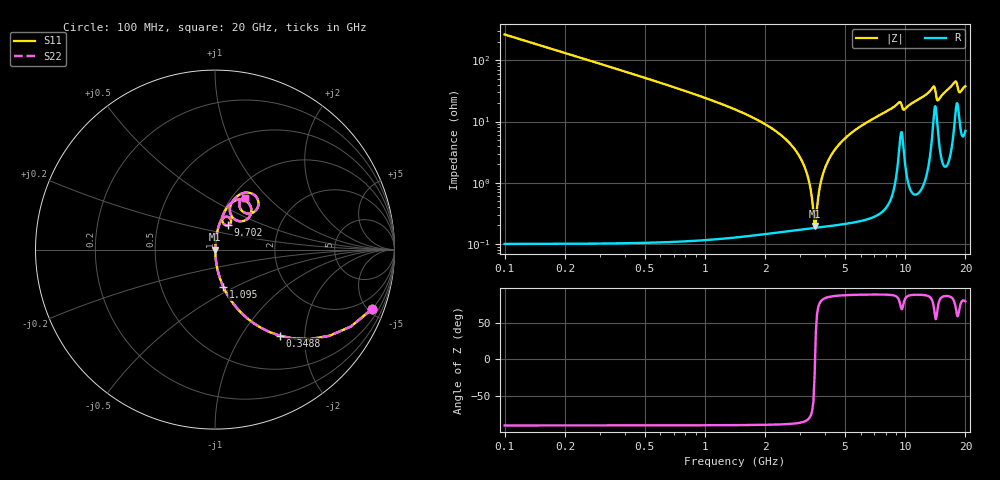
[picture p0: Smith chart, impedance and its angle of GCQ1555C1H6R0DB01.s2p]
!Murata Part Number: GCQ1555C1H6R0DB01
!These Parameters are Measured in Series Mode Connection
!Data Generated on Jan 08, 2026
!  o--ll--o
!Port1  Port2
!  o------o
!Operation Temp=25[degC], DC Bias Voltage=0[V]
!Freq. Start=100[MHz] Stop=20[GHz] 401[Steps]
# Hz S RI R 50
!Freq.(Hz) S11(Real) S11(Imag) S21(Real) S21(Imag) S12(Real) S12(Imag) S22(Real) S22(Imag)
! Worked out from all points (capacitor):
!   401 points, 100 MHz to 20 GHz, reference 50 ohm
!   read as one part in series: C = 6 pF near 199.5 MHz
!   lowest |Z| = 196 mohm at 3.533 GHz (marker M1)
!   series resonance near 3.55 GHz, so ESL is about 340 pH
!   S11 on the Smith chart (normalised r, x): 100 MHz: 1.00, -5.30; 348.8 MHz: 1.00, -1.51; 1.095 GHz: 1.00, -0.44; 9.702 GHz: 1.11, +0.31; 20 GHz: 1.14, +0.74
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1e8  0.8753 -0.3302  0.1247 0.3302  0.1247 0.3302  0.8753 -0.3302
3.4875e8  0.3621 -0.4799  0.6379 0.4799  0.6379 0.4799  0.3621 -0.4799
6.4725e8  0.1363 -0.3418  0.8637 0.3418  0.8637 0.3418  0.1363 -0.3418
1.095e9  0.0468 -0.2086  0.9532 0.2086  0.9532 0.2086  0.0468 -0.2086
2.83625e9  0.0028 -0.0337  0.9972 0.0337  0.9972 0.0337  0.0028 -0.0337
3.23425e9  0.00195 -0.0139  0.9981 0.0139  0.9981 0.0139  0.00195 -0.0139
3.43325e9  0.00182 -0.00498  0.9982 0.00498  0.9982 0.00498  0.00182 -0.00498
3.53275e9  0.00182 -0.000717  0.9982 0.000717  0.9982 0.000717  0.00182 -0.000717
3.63225e9  0.00185 0.00343  0.9982 -0.00343  0.9982 -0.00343  0.00185 0.00343
3.93075e9  0.00213 0.0153  0.9979 -0.0153  0.9979 -0.0153  0.00213 0.0153
4.3785e9  0.00299 0.0316  0.997 -0.0316  0.997 -0.0316  0.00299 0.0316
6.7665e9  0.0137 0.1047  0.9863 -0.1047  0.9863 -0.1047  0.0137 0.1047
9.30375e9  0.065 0.1831  0.935 -0.1831  0.935 -0.1831  0.065 0.1831
9.70175e9  0.073 0.1364  0.927 -0.1364  0.927 -0.1364  0.073 0.1364
1.005e10  0.0421 0.1537  0.9579 -0.1537  0.9579 -0.1537  0.0421 0.1537
1.338325e10  0.1153 0.2745  0.8847 -0.2745  0.8847 -0.2745  0.1153 0.2745
1.39305e10  0.1922 0.2522  0.8078 -0.2522  0.8078 -0.2522  0.1922 0.2522
1.45275e10  0.1064 0.1706  0.8936 -0.1706  0.8936 -0.1706  0.1064 0.1706
1.67165e10  0.1302 0.3022  0.8698 -0.3022  0.8698 -0.3022  0.1302 0.3022
1.7811e10  0.2273 0.2962  0.7727 -0.2962  0.7727 -0.2962  0.2273 0.2962
1.865675e10  0.1525 0.2137  0.8475 -0.2137  0.8475 -0.2137  0.1525 0.2137
2e10  0.1659 0.2888  0.8341 -0.2888  0.8341 -0.2888  0.1659 0.2888
